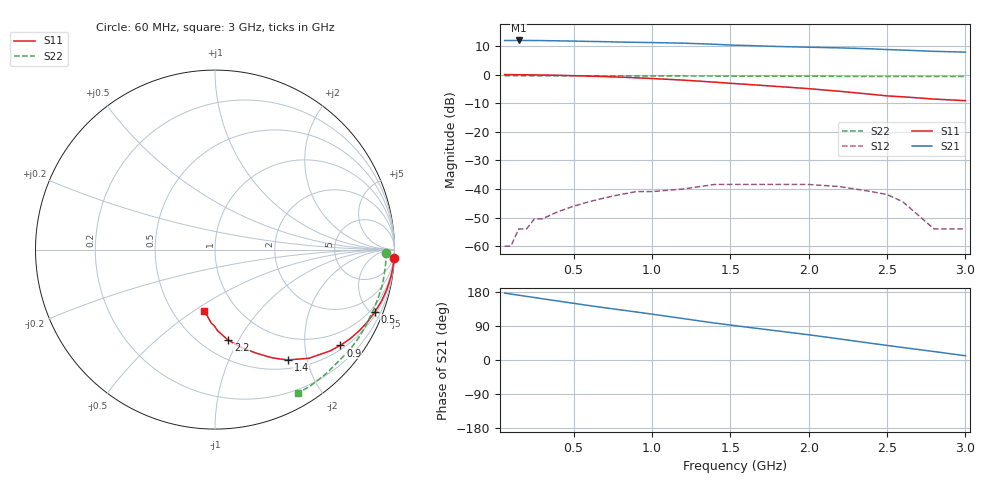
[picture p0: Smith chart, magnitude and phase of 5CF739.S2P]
!CF739, Dual Gate GaAs FET in SOT143 package
!V DS = 5V, I D = 15 mA, Vg2 = 2V
# GHZ S MA R 50
!f GHz  S11  S21  S12  S22
!  MAG  ANG  MAG  ANG  MAG  ANG  MAG  ANG
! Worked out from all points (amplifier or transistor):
!   26 points, 60 MHz to 3 GHz, reference 50 ohm
!   highest |S21| = 11.9 dB at 150 MHz (marker M1)
!   |S21| within 3 dB of that: start of sweep to 2.429 GHz
!   unconditionally stable (mu >= 1): 1.376 GHz to end of sweep
!   at 200 MHz: K = 0.17, MSG = 33.0 dB, |S12| = -54.0 dB
!   at 1 GHz: K = 0.73, MSG = 26.1 dB, |S12| = -40.9 dB
!   at 3 GHz: K = 12.75, MAG = 16.9 dB, |S12| = -54.0 dB
!   S11 on the Smith chart (normalised r, x): 60 MHz: 1, -44; 500 MHz: 0.65, -5.24; 900 MHz: 0.60, -2.84; 1.4 GHz: 0.63, -1.68; 2.2 GHz: 0.66, -0.91; 3 GHz: 0.70, -0.55
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0.06  0.999 -2.6  3.94 176.6  0.001 78.1  0.955 -1.0
0.1  0.998 -4.3  3.94 174.0  0.001 86.2  0.955 -1.8
0.15  0.995 -6.6  3.95 171.0  0.002 82.8  0.954 -2.6
0.2  0.992 -8.7  3.95 167.9  0.002 85.5  0.954 -3.4
0.25  0.987 -10.8  3.94 164.9  0.003 85.5  0.954 -4.3
0.3  0.983 -13.0  3.93 161.7  0.003 84.6  0.954 -5.2
0.5  0.956 -21.3  3.85 149.6  0.005 78.2  0.953 -8.6
0.6  0.94 -25.4  3.8 143.6  0.006 76.7  0.953 -10.3
0.7  0.922 -29.4  3.76 137.8  0.007 75.8  0.953 -12.1
0.9  0.879 -37.4  3.66 126.7  0.009 70.0  0.949 -15.5
1  0.854 -41.4  3.63 121.0  0.009 69.5  0.947 -17.1
1.2  0.8 -49.2  3.54 109.3  0.01 66.4  0.945 -20.8
1.4  0.737 -56.5  3.39 97.5  0.012 60.7  0.941 -24.5
1.6  0.676 -62.7  3.23 87.0  0.012 55.0  0.94 -28.1
1.8  0.62 -68.4  3.1 76.8  0.012 52.7  0.939 -31.7
2  0.567 -74.6  3.01 66.6  0.012 48.1  0.936 -35.6
2.2  0.51 -81.7  2.93 55.5  0.011 42.8  0.93 -39.9
2.4  0.452 -88.2  2.82 44.0  0.009 36.9  0.927 -44.9
2.5  0.424 -90.6  2.74 38.5  0.008 35.3  0.928 -47.5
2.6  0.409 -93.0  2.68 33.0  0.006 30.4  0.927 -50.2
2.8  0.373 -96.5  2.55 22.3  0.002 16.6  0.927 -55.3
3  0.35 -100.1  2.47 11.2  0.002 -129.4  0.924 -59.9
